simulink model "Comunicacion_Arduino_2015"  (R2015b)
settings: Solver=VariableStepAuto  SolverMode=SingleTasking  StartTime=0.0  StopTime=60  RelTol=1e-3
undefined symbols (not defined in the file or in its folder): LF, serial
libraries: instrumentlib x3

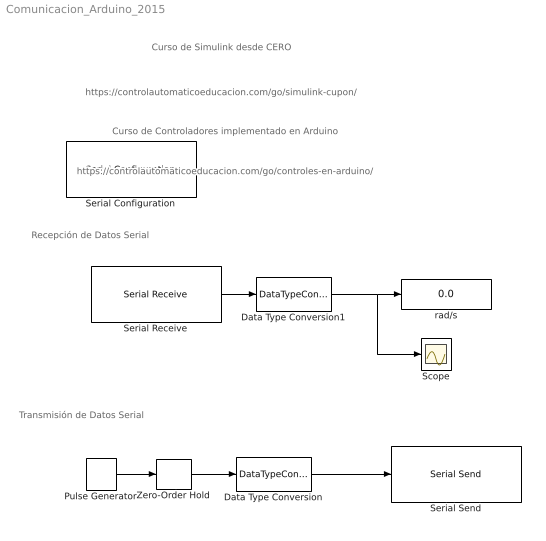
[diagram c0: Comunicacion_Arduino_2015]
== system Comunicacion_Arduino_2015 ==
  note: Transmisión de Datos Serial
  note: Recepción de Datos Serial
  note: Curso de Simulink desde CERO
  note: https://controlautomaticoeducacion.com/go/simulink-cupon/
  note: https://controlautomaticoeducacion.com/go/controles-en-arduino/
  note: Curso de Controladores implementado en Arduino
  Data Type Conversion : DataTypeConversion  OutDataTypeStr=single
  Data Type Conversion1 : DataTypeConversion  OutDataTypeStr=double
  Pulse Generator : DiscretePulseGenerator  PulseType=Time based  Amplitude=5  Period=4  PulseWidth=50
  Scope : Scope
  Serial Configuration : instrumentlib/Serial Configuration  Priority=-200000  ObjConstructor=serial('COM1');  ComPortMenu=COM1  ComPort=COM1  BaudRate=9600  DataBits=8  Parity=none  StopBits=1  ByteOrder=LittleEndian  FlowControl=none  Timeout=10
  Serial Receive : instrumentlib/Serial Receive  Priority=1  ObjConstructor=serial('COM1');  ComPortMenu=COM1  ComPort=COM1  DataType=single  Terminator=LF ('\n')  DataSize=[1 1]  EnableBlockingMode=on  ActionDataUnavailable=Output last received value  CustomValue=0  SampleTime=0.05
  Serial Send : instrumentlib/Serial Send  Priority=1  ObjConstructor=serial('COM1');  ComPortMenu=COM1  ComPort=COM1  Terminator=<none>  EnableBlockingMode=on
  Zero-Order Hold : ZeroOrderHold  SampleTime=0.05
  rad/s : Display
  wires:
  Pulse Generator/1 -> Zero-Order Hold/1
  Zero-Order Hold/1 -> Data Type Conversion/1
  Data Type Conversion/1 -> Serial Send/1
  Serial Receive/1 -> Data Type Conversion1/1
  Data Type Conversion1/1 -> Scope/1, rad/s/1
